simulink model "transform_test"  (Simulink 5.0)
settings: Solver=ode45  StartTime=0.0  StopTime=10.0  RelTol=1e-3
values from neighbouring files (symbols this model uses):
  a1 = 8.5    [startup.m]
  a2 = 48    [startup.m]
  a3 = 38+11/16    (= 38.6875)    [startup.m]
  a4 = 18.5    [startup.m]
  R1A = 10    [startup.m]
  R1B = 35.875    [startup.m]
  R2C = 36    [startup.m]
  R2D = 9+7/8    (= 9.875)    [startup.m]
  R3F = 4.5    [startup.m]
  R3G = 5.5    [startup.m]
  REF = 29.625    [startup.m]
  RFH = 9.5    [startup.m]
  RGH = 9.5    [startup.m]
  T01A = acos(RAJ/R1A)    [startup.m]
  T12C = acos((a2^2 + R2C^2 - R1C^2)/(2*a2*R2C))    [startup.m]
  T23D = 0.1317    [startup.m]
  TB12 = acos((R1B^2 + a2^2 - R2B^2)/(2*a2*R1B))    [startup.m]
  TD23 = acos((R2D^2 + a3^2 - R3D^2)/(2*a3*R2D))    [startup.m]
  TDFE = 0.0503    [startup.m]
  TG34 = 1.6966    [startup.m]
libraries: simulink x2

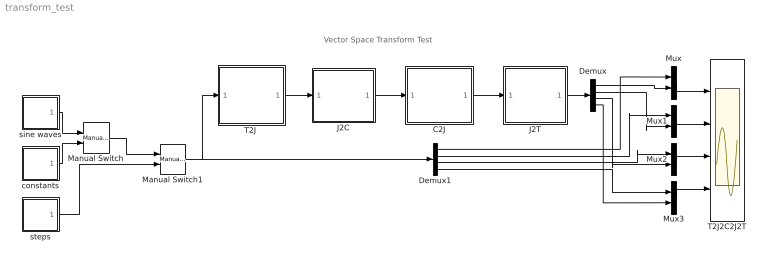
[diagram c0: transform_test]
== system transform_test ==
  note: Vector Space Transform Test
  C2J : Subsystem
  Demux : Demux
  Demux1 : Demux
  J2C : Subsystem
  J2T : Subsystem
  Manual Switch : simulink/Signal Routing/Manual Switch  sw=1  action=0
  Manual Switch1 : simulink/Signal Routing/Manual Switch  sw=1  action=0
  Mux{,1..3} (4 alike) : Mux  Inputs=2
  "T2J " : Subsystem
  T2J2C2J2T : Scope  NumInputPorts=4
  constants : Subsystem
  sine waves : Subsystem
  steps : Subsystem
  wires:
  Mux/1 -> T2J2C2J2T/1
  Mux1/1 -> T2J2C2J2T/2
  Mux2/1 -> T2J2C2J2T/3
  Mux3/1 -> T2J2C2J2T/4
  Demux1/1 -> Mux/1
  Demux1/2 -> Mux1/1
  Demux1/3 -> Mux2/1
  Demux1/4 -> Mux3/1
  Demux/1 -> Mux/2
  Demux/2 -> Mux1/2
  Demux/3 -> Mux2/2
  Demux/4 -> Mux3/2
  sine waves/1(ref) -> Manual Switch/1
  constants/1(ref) -> Manual Switch/2
  steps/1(ref) -> Manual Switch1/2
  Manual Switch/1 -> Manual Switch1/1
  Manual Switch1/1 -> Demux1/1, "T2J "/1(yp)
  J2C/1(ycdes) -> C2J/1(yc)
  "T2J "/1(qdes) -> J2C/1(qdes)
  C2J/1(q) -> J2T/1(q)
  J2T/1(yb) -> Demux/1

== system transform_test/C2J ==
  note: Swing
  note: q1
  note: Cylinder to Joint Transformation
  yc : Inport
  Boom : Subsystem
  Bucket : Subsystem
  Demux : Demux
  Mux : Mux
  Stick : Subsystem
  q : Outport
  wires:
  Mux/1 -> q/1
  yc/1 -> Demux/1
  Boom/1(q2) -> Mux/2
  Demux/2 -> Boom/1(yc3)
  Demux/1 -> Mux/1
  Demux/3 -> Stick/1(yc4)
  Stick/1(q3) -> Mux/3
  Demux/4 -> Bucket/1(yc5)
  Bucket/1(q4) -> Mux/4

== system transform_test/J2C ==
  note: Joint Space -> Cylinder Space Transformation
  note: Swing Cylinders
  qdes : Inport
  Boom cylinder : Subsystem
  Bucket cylinder : Subsystem
  Demux : Demux
  Mux : Mux
  Stick cylinder : Subsystem
  overswing  protection : Saturate  UpperLimit=pi/3  LowerLimit=-pi/2
  ycdes : Outport
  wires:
  qdes/1 -> Demux/1
  Mux/1 -> ycdes/1
  Demux/2 -> Boom cylinder/1(q2)
  Boom cylinder/1(yc3) -> Mux/2
  Demux/3 -> Stick cylinder/1(q3)
  Stick cylinder/1(yc4) -> Mux/3
  Demux/4 -> Bucket cylinder/1(q4)
  Bucket cylinder/1(yc5) -> Mux/4
  Demux/1 -> overswing  protection/1
  overswing  protection/1 -> Mux/1

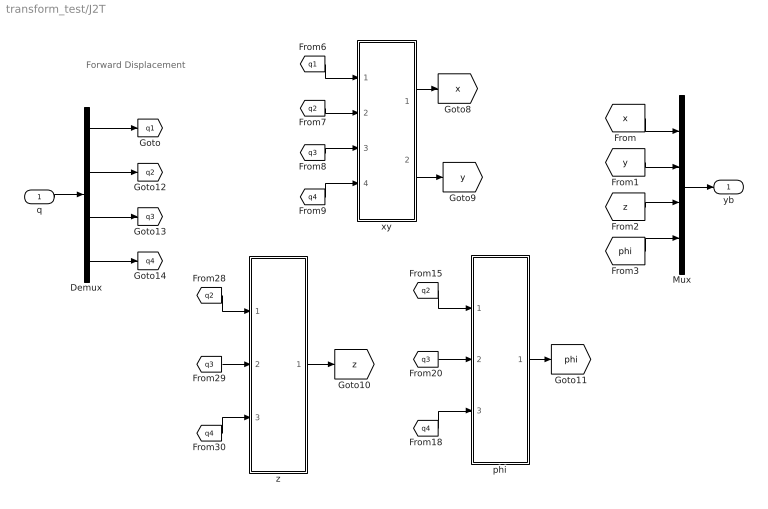
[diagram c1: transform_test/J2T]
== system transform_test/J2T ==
  note: Forward Displacement
  q : Inport
  Demux : Demux
  Mux : Mux
  phi : Subsystem
  xy : Subsystem
  z : Subsystem
  yb : Outport
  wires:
  [q2] -> z/1(q2)
  [q3] -> z/2(q3)
  [q4] -> z/3(q4)
  z/1(z) -> [z]
  q/1 -> Demux/1
  Demux/2 -> [q2]
  Demux/1 -> [q1]
  Demux/3 -> [q3]
  Demux/4 -> [q4]
  [q2] -> phi/1(q2)
  [q3] -> phi/2(q3)
  phi/1(phi) -> [phi]
  Mux/1 -> yb/1
  [x] -> Mux/1
  [y] -> Mux/2
  [z] -> Mux/3
  [phi] -> Mux/4
  xy/1(x) -> [x]
  [q1] -> xy/1(q1)
  [q2] -> xy/2(q2)
  [q3] -> xy/3(q3)
  [q4] -> xy/4(q4)
  [q4] -> phi/3(q4)
  xy/2(y) -> [y]

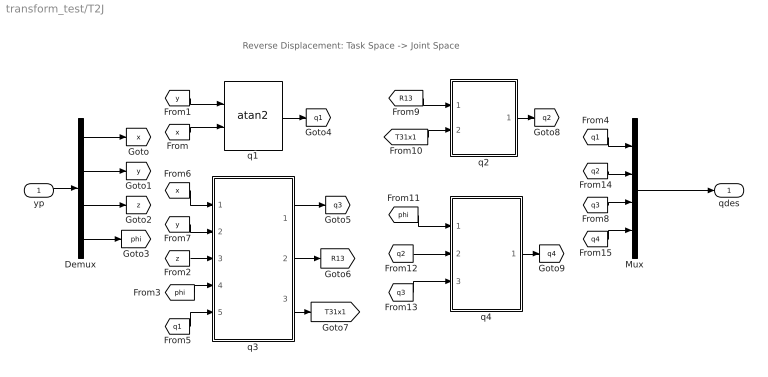
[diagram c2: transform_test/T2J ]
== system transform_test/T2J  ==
  note: Reverse Displacement: Task Space -> Joint Space
  yp : Inport
  Demux : Demux
  Mux : Mux
  q1 : Trigonometry  Operator=atan2
  q2 : Subsystem
  q3 : Subsystem
  q4 : Subsystem
  qdes : Outport
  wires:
  [x] -> q3/1(x)
  [y] -> q3/2(y)
  [z] -> q3/3(z)
  [phi] -> q3/4(phi)
  [q1] -> q3/5(q1)
  q3/1(q3) -> [q3]
  q3/2(R13) -> [R13]
  [y] -> q1/1
  [x] -> q1/2
  q1/1 -> [q1]
  q3/3(T31x1) -> [T31x1]
  [R13] -> q2/1(R13)
  [T31x1] -> q2/2(T31x1)
  [q3] -> q4/3(q3)
  [q2] -> q4/2(q2)
  [phi] -> q4/1(phi)
  q2/1(q2) -> [q2]
  q4/1(q4) -> [q4]
  Mux/1 -> qdes/1
  [q1] -> Mux/1
  [q3] -> Mux/3
  [q2] -> Mux/2
  [q4] -> Mux/4
  yp/1 -> Demux/1
  Demux/1 -> [x]
  Demux/2 -> [y]
  Demux/3 -> [z]
  Demux/4 -> [phi]

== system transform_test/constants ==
  DOF1 : Constant  Value=60
  DOF2 : Constant  Value=0
  DOF3 : Constant  Value=3
  DOF4 : Constant  Value=5*pi/6
  Mux2 : Mux
  ref : Outport
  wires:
  Mux2/1 -> ref/1
  DOF1/1 -> Mux2/1
  DOF2/1 -> Mux2/2
  DOF3/1 -> Mux2/3
  DOF4/1 -> Mux2/4

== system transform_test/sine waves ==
  DOF1 : Sin  Amplitude=4  Bias=46  Frequency=2*pi*0.1  SampleTime=0
  DOF2 : Sin  Amplitude=2  Frequency=2*pi*0.1  SampleTime=0
  DOF3 : Sin  Amplitude=6  Bias=3  Frequency=2*pi*0.1  SampleTime=0
  DOF4 : Sin  Amplitude=0.2  Bias=5*pi/6  Frequency=2*pi*0.1  SampleTime=0
  Mux2 : Mux
  ref : Outport
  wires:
  DOF1/1 -> Mux2/1
  DOF4/1 -> Mux2/4
  DOF3/1 -> Mux2/3
  DOF2/1 -> Mux2/2
  Mux2/1 -> ref/1

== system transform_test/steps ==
  Constant : Constant  Value=[46 0 3 5*pi/6]
  DOF1 : Step  Time=0.25  SampleTime=0
  DOF2 : Step  Time=0.5  After=0.5  SampleTime=0
  DOF3 : Step  Time=.75  After=-.5  SampleTime=0
  DOF4 : Step  After=-1  SampleTime=0
  Mux2 : Mux
  Sum : Sum  Inputs=|++
  ref : Outport
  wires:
  DOF1/1 -> Mux2/1
  DOF4/1 -> Mux2/4
  DOF3/1 -> Mux2/3
  DOF2/1 -> Mux2/2
  Mux2/1 -> Sum/1
  Sum/1 -> ref/1
  Constant/1 -> Sum/2

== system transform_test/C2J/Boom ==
  note: TA1B
  yc3 : Inport
  CosineLawA : Subsystem
  R1A : Constant  Value=R1A
  R1B : Constant  Value=R1B
  Sum : Sum  Inputs=+---
  T01A : Constant  Value=T01A
  TA1B : Constant  Value=TB12
  pi : Constant  Value=pi
  q2 : Outport
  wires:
  pi/1 -> Sum/1
  T01A/1 -> Sum/2
  TA1B/1 -> Sum/4
  CosineLawA/1(theta) -> Sum/3
  R1A/1 -> CosineLawA/1(r1)
  R1B/1 -> CosineLawA/2(r2)
  Sum/1 -> q2/1
  yc3/1 -> CosineLawA/3(r3)

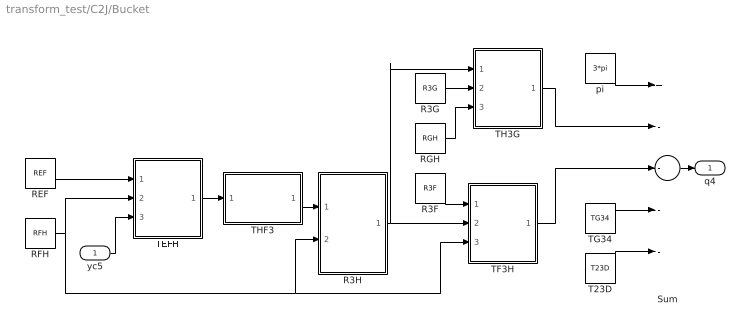
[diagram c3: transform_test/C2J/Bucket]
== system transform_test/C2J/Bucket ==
  yc5 : Inport
  R3F : Constant  Value=R3F
  R3G : Constant  Value=R3G
  R3H : Subsystem
  REF : Constant  Value=REF
  RFH : Constant  Value=RFH
  RGH : Constant  Value=RGH
  Sum : Sum  Inputs=+----
  T23D : Constant  Value=T23D
  TEFH : Subsystem
  TF3H : Subsystem
  TG34 : Constant  Value=TG34
  TH3G : Subsystem
  THF3 : Subsystem
  pi : Constant  Value=3*pi
  q4 : Outport
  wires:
  TEFH/1(TEFH) -> THF3/1(TEFH)
  REF/1 -> TEFH/1(r1)
  yc5/1 -> TEFH/3(r3)
  RFH/1 -> TEFH/2(r2), R3H/2(RFH), TF3H/3(r3)
  THF3/1(THF3) -> R3H/1(THF3)
  R3F/1 -> TF3H/1(r1)
  R3H/1(R3H) -> TF3H/2(r2), TH3G/1(r1)
  R3G/1 -> TH3G/2(r2)
  RGH/1 -> TH3G/3(r3)
  pi/1 -> Sum/1
  Sum/1 -> q4/1
  T23D/1 -> Sum/5
  TG34/1 -> Sum/4
  TH3G/1(TH3G) -> Sum/2
  TF3H/1(TF3H) -> Sum/3

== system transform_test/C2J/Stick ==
  note: TC2D
  yc4 : Inport
  CosineLawA : Subsystem
  R2C : Constant  Value=R2C
  R2D : Constant  Value=R2D
  Sum : Sum  Inputs=+---
  T12C : Constant  Value=T12C
  TD23 : Constant  Value=TD23
  pi : Constant  Value=3*pi
  q3 : Outport
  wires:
  pi/1 -> Sum/1
  T12C/1 -> Sum/2
  TD23/1 -> Sum/4
  CosineLawA/1(theta) -> Sum/3
  R2C/1 -> CosineLawA/1(r1)
  R2D/1 -> CosineLawA/2(r2)
  Sum/1 -> q3/1
  yc4/1 -> CosineLawA/3(r3)

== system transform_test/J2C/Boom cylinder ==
  q2 : Inport
  Constant : Constant  Value=pi
  Constant1 : Constant  Value=T01A
  Constant2 : Constant  Value=TB12
  CosineLawB : Subsystem
  Sum : Sum  Inputs=+---
  yc3 : Outport
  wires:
  Constant/1 -> Sum/1
  Constant1/1 -> Sum/2
  Sum/1 -> CosineLawB/1(TA1B)
  CosineLawB/1(yc3) -> yc3/1
  q2/1 -> Sum/3
  Constant2/1 -> Sum/4

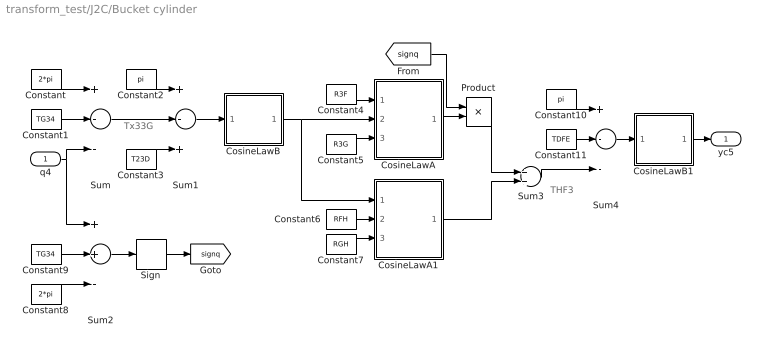
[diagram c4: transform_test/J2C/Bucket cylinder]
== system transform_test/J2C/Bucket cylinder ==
  note: Tx33G
  note: THF3
  q4 : Inport
  Constant : Constant  Value=2*pi
  Constant1 : Constant  Value=TG34
  Constant10 : Constant  Value=pi
  Constant11 : Constant  Value=TDFE
  Constant2 : Constant  Value=pi
  Constant3 : Constant  Value=T23D
  Constant4 : Constant  Value=R3F
  Constant5 : Constant  Value=R3G
  Constant6 : Constant  Value=RFH
  Constant7 : Constant  Value=RGH
  Constant8 : Constant  Value=2*pi
  Constant9 : Constant  Value=TG34
  CosineLawA : Subsystem
  CosineLawA1 : Subsystem
  CosineLawB : Subsystem
  CosineLawB1 : Subsystem
  Product : Product
  Sign : Signum
  Sum : Sum  Inputs=+--
  Sum1 : Sum  Inputs=+-+
  Sum2 : Sum  Inputs=++-
  Sum3 : Sum
  Sum4 : Sum  Inputs=+--
  yc5 : Outport
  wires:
  Constant/1 -> Sum/1
  Constant1/1 -> Sum/2
  Sum/1 -> Sum1/2
  Constant2/1 -> Sum1/1
  Constant3/1 -> Sum1/3
  Sum1/1 -> CosineLawB/1(TG3F)
  CosineLawB/1(rFG) -> CosineLawA/2(r2), CosineLawA1/1(r1)
  Constant4/1 -> CosineLawA/1(r1)
  Constant5/1 -> CosineLawA/3(r3)
  Constant6/1 -> CosineLawA1/2(r2)
  Constant7/1 -> CosineLawA1/3(r3)
  Constant9/1 -> Sum2/2
  Constant8/1 -> Sum2/3
  Sum2/1 -> Sign/1
  [signq] -> Product/1
  CosineLawA/1(T3FG) -> Product/2
  Sign/1 -> [signq]
  Product/1 -> Sum3/1
  CosineLawA1/1(THFG) -> Sum3/2
  Constant10/1 -> Sum4/1
  Sum3/1 -> Sum4/3
  Constant11/1 -> Sum4/2
  Sum4/1 -> CosineLawB1/1(TEFH)
  CosineLawB1/1(yc5) -> yc5/1
  q4/1 -> Sum/3, Sum2/1

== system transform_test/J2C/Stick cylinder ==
  q3 : Inport
  Constant : Constant  Value=pi
  Constant1 : Constant  Value=TD23
  Constant2 : Constant  Value=T12C
  CosineLawB : Subsystem
  Sum : Sum  Inputs=+---
  yc4 : Outport
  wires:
  Constant/1 -> Sum/1
  Constant1/1 -> Sum/2
  Sum/1 -> CosineLawB/1(TC2D)
  CosineLawB/1(yc4) -> yc4/1
  q3/1 -> Sum/3
  Constant2/1 -> Sum/4

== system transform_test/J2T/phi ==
  q2 : Inport
  q3 : Inport  Port=2
  q4 : Inport  Port=3
  Constant : Constant  Value=3*pi
  Sum : Sum  Inputs=+++-
  phi : Outport
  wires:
  q2/1 -> Sum/1
  q3/1 -> Sum/2
  q4/1 -> Sum/3
  Constant/1 -> Sum/4
  Sum/1 -> phi/1

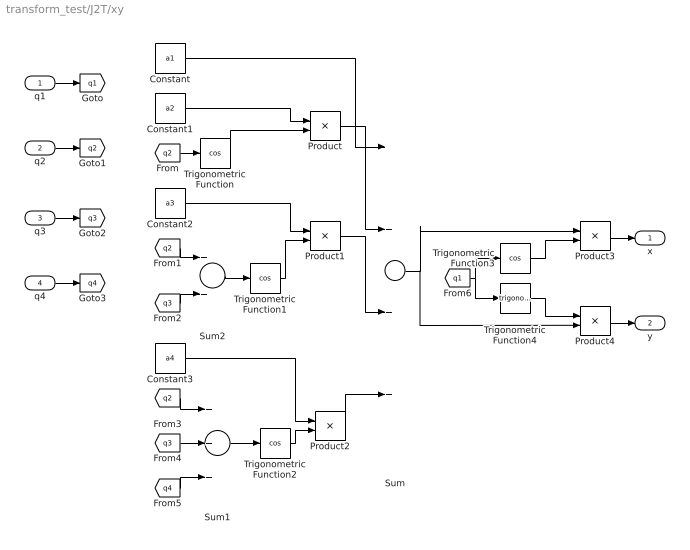
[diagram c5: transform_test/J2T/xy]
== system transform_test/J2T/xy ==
  q1 : Inport
  q2 : Inport  Port=2
  q3 : Inport  Port=3
  q4 : Inport  Port=4
  Constant : Constant  Value=a1
  Constant1 : Constant  Value=a2
  Constant2 : Constant  Value=a3
  Constant3 : Constant  Value=a4
  Product{,1..4} (5 alike) : Product
  Sum : Sum  Inputs=++++
  Sum1 : Sum  Inputs=+++
  Sum2 : Sum
  Trigonometric Function{,1..3} (4 alike) : Trigonometry  Operator=cos
  Trigonometric Function4 : Trigonometry
  x : Outport
  y : Outport  Port=2
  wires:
  q1/1 -> [q1]
  q2/1 -> [q2]
  q3/1 -> [q3]
  q4/1 -> [q4]
  Constant/1 -> Sum/1
  Product/1 -> Sum/2
  Constant1/1 -> Product/1
  [q3] -> Sum2/2
  [q2] -> Sum2/1
  Constant2/1 -> Product1/1
  Product1/1 -> Sum/3
  Product2/1 -> Sum/4
  Constant3/1 -> Product2/1
  [q2] -> Sum1/1
  [q3] -> Sum1/2
  [q4] -> Sum1/3
  Product3/1 -> x/1
  Sum/1 -> Product4/2, Product3/1
  Trigonometric Function/1 -> Product/2
  [q2] -> Trigonometric Function/1
  Sum2/1 -> Trigonometric Function1/1
  Trigonometric Function1/1 -> Product1/2
  Sum1/1 -> Trigonometric Function2/1
  Trigonometric Function2/1 -> Product2/2
  Product4/1 -> y/1
  Trigonometric Function3/1 -> Product3/2
  [q1] -> Trigonometric Function3/1, Trigonometric Function4/1
  Trigonometric Function4/1 -> Product4/1

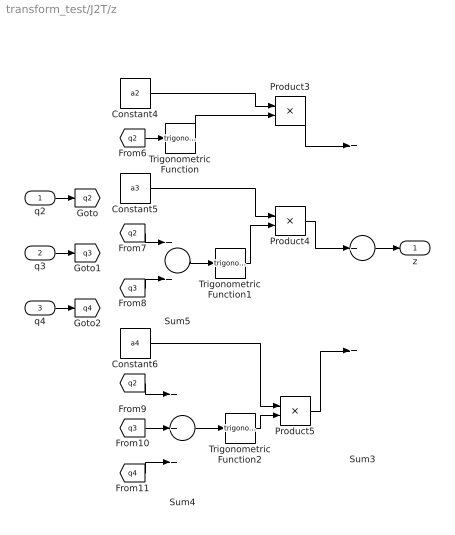
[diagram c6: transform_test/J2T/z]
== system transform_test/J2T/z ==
  q2 : Inport
  q3 : Inport  Port=2
  q4 : Inport  Port=3
  Constant4 : Constant  Value=a2
  Constant5 : Constant  Value=a3
  Constant6 : Constant  Value=a4
  Product3 : Product
  Product4 : Product
  Product5 : Product
  Sum3 : Sum  Inputs=+++
  Sum4 : Sum  Inputs=+++
  Sum5 : Sum
  Trigonometric Function : Trigonometry
  Trigonometric Function1 : Trigonometry
  Trigonometric Function2 : Trigonometry
  z : Outport
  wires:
  q3/1 -> [q3]
  q4/1 -> [q4]
  q2/1 -> [q2]
  Constant4/1 -> Product3/1
  [q3] -> Sum5/2
  [q2] -> Sum5/1
  Constant5/1 -> Product4/1
  Constant6/1 -> Product5/1
  [q2] -> Sum4/1
  [q3] -> Sum4/2
  [q4] -> Sum4/3
  Trigonometric Function/1 -> Product3/2
  [q2] -> Trigonometric Function/1
  Sum5/1 -> Trigonometric Function1/1
  Trigonometric Function1/1 -> Product4/2
  Sum4/1 -> Trigonometric Function2/1
  Trigonometric Function2/1 -> Product5/2
  Product3/1 -> Sum3/1
  Product4/1 -> Sum3/2
  Product5/1 -> Sum3/3
  Sum3/1 -> z/1

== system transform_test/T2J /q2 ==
  note: T213
  R13 : Inport
  T31x1 : Inport  Port=2
  CosineLawA : Subsystem
  Sum : Sum  Inputs=|++
  a2 : Constant  Value=a2
  a3 : Constant  Value=a3
  q2 : Outport
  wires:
  a2/1 -> CosineLawA/1(r1)
  a3/1 -> CosineLawA/3(r3)
  CosineLawA/1(theta) -> Sum/1
  Sum/1 -> q2/1
  R13/1 -> CosineLawA/2(r2)
  T31x1/1 -> Sum/2

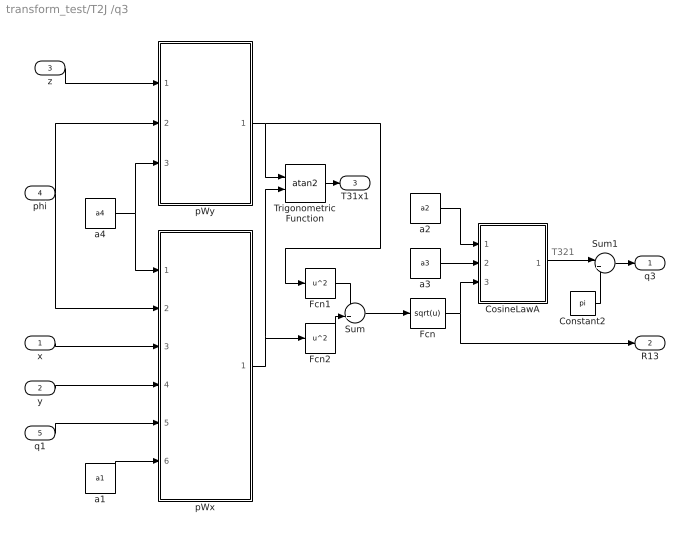
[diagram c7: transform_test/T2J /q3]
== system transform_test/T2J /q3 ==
  note: T321
  x : Inport
  y : Inport  Port=2
  z : Inport  Port=3
  phi : Inport  Port=4
  q1 : Inport  Port=5
  Constant2 : Constant  Value=pi
  CosineLawA : Subsystem
  Fcn : Fcn  Expr=sqrt(u)
  Fcn1 : Fcn  Expr=u^2
  Fcn2 : Fcn  Expr=u^2
  Sum : Sum
  Sum1 : Sum  Inputs=|++
  Trigonometric Function : Trigonometry  Operator=atan2
  a1 : Constant  Value=a1
  a2 : Constant  Value=a2
  a3 : Constant  Value=a3
  a4 : Constant  Value=a4
  pWx : Subsystem
  pWy : Subsystem
  q3 : Outport
  R13 : Outport  Port=2
  T31x1 : Outport  Port=3
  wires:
  a1/1 -> pWx/6(a1)
  q1/1 -> pWx/5(q1)
  y/1 -> pWx/4(y)
  x/1 -> pWx/3(x)
  a4/1 -> pWx/1(a4), pWy/3(a4)
  z/1 -> pWy/1(z)
  phi/1 -> pWx/2(phi), pWy/2(phi)
  pWy/1(pWy) -> Fcn1/1, Trigonometric Function/1
  Trigonometric Function/1 -> T31x1/1
  Fcn1/1 -> Sum/1
  Fcn2/1 -> Sum/2
  Sum/1 -> Fcn/1
  pWx/1(pWx) -> Fcn2/1, Trigonometric Function/2
  a3/1 -> CosineLawA/2(r2)
  a2/1 -> CosineLawA/1(r1)
  Fcn/1 -> CosineLawA/3(r3), R13/1
  Sum1/1 -> q3/1
  Constant2/1 -> Sum1/2
  CosineLawA/1(theta) -> Sum1/1

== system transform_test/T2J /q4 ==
  phi : Inport
  q2 : Inport  Port=2
  q3 : Inport  Port=3
  Constant : Constant  Value=3*pi
  Sum : Sum  Inputs=+--+
  q4 : Outport
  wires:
  phi/1 -> Sum/1
  q2/1 -> Sum/2
  Sum/1 -> q4/1
  q3/1 -> Sum/3
  Constant/1 -> Sum/4

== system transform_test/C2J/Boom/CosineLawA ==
  r1 : Inport
  r2 : Inport  Port=2
  r3 : Inport  Port=3
  Fcn1 : Fcn  Expr=u^2
  Fcn2 : Fcn  Expr=u^2
  Fcn3 : Fcn  Expr=u^2
  Gain : Gain  Gain=2
  Product : Product
  Product1 : Product  Inputs=*/
  Sum : Sum  Inputs=++-
  Trigonometric Function : Trigonometry  Operator=acos
  theta : Outport
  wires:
  r3/1 -> Fcn3/1
  Fcn1/1 -> Sum/1
  Fcn2/1 -> Sum/2
  Fcn3/1 -> Sum/3
  r2/1 -> Fcn2/1, Product/1
  r1/1 -> Fcn1/1, Product/2
  Product/1 -> Gain/1
  Sum/1 -> Product1/1
  Gain/1 -> Product1/2
  Product1/1 -> Trigonometric Function/1
  Trigonometric Function/1 -> theta/1

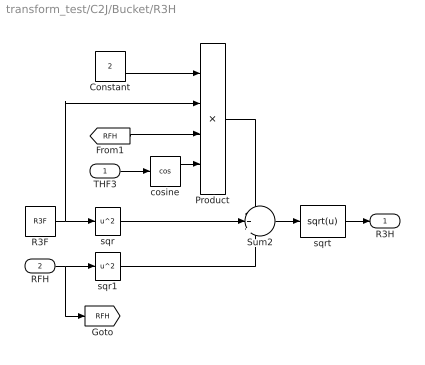
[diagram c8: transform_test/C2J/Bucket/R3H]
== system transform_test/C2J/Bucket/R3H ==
  THF3 : Inport
  RFH : Inport  Port=2
  Constant : Constant  Value=2
  Product : Product  Inputs=4
  R3F : Constant  Value=R3F
  Sum2 : Sum  Inputs=-++
  cosine : Trigonometry  Operator=cos
  sqr : Fcn  Expr=u^2
  sqr1 : Fcn  Expr=u^2
  sqrt : Fcn  Expr=sqrt(u)
  R3H : Outport
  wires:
  R3F/1 -> sqr/1, Product/2
  sqr1/1 -> Sum2/3
  Constant/1 -> Product/1
  [RFH] -> Product/3
  sqr/1 -> Sum2/2
  Product/1 -> Sum2/1
  cosine/1 -> Product/4
  Sum2/1 -> sqrt/1
  THF3/1 -> cosine/1
  sqrt/1 -> R3H/1
  RFH/1 -> sqr1/1, [RFH]

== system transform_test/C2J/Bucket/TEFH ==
  r1 : Inport
  r2 : Inport  Port=2
  r3 : Inport  Port=3
  Fcn1 : Fcn  Expr=u^2
  Fcn2 : Fcn  Expr=u^2
  Fcn3 : Fcn  Expr=u^2
  Gain : Gain  Gain=2
  Product : Product
  Product1 : Product  Inputs=*/
  Sum : Sum  Inputs=++-
  Trigonometric Function : Trigonometry  Operator=acos
  TEFH : Outport
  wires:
  r3/1 -> Fcn3/1
  Fcn1/1 -> Sum/1
  Fcn2/1 -> Sum/2
  Fcn3/1 -> Sum/3
  r2/1 -> Fcn2/1, Product/1
  r1/1 -> Fcn1/1, Product/2
  Product/1 -> Gain/1
  Sum/1 -> Product1/1
  Gain/1 -> Product1/2
  Product1/1 -> Trigonometric Function/1
  Trigonometric Function/1 -> TEFH/1

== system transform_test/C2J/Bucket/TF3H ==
  r1 : Inport
  r2 : Inport  Port=2
  r3 : Inport  Port=3
  Fcn1 : Fcn  Expr=u^2
  Fcn2 : Fcn  Expr=u^2
  Fcn3 : Fcn  Expr=u^2
  Gain : Gain  Gain=2
  Product : Product
  Product1 : Product  Inputs=*/
  Sum : Sum  Inputs=++-
  Trigonometric Function : Trigonometry  Operator=acos
  TF3H : Outport
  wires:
  r3/1 -> Fcn3/1
  Fcn1/1 -> Sum/1
  Fcn2/1 -> Sum/2
  Fcn3/1 -> Sum/3
  r2/1 -> Fcn2/1, Product/1
  r1/1 -> Fcn1/1, Product/2
  Product/1 -> Gain/1
  Sum/1 -> Product1/1
  Gain/1 -> Product1/2
  Product1/1 -> Trigonometric Function/1
  Trigonometric Function/1 -> TF3H/1

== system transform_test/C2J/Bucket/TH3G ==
  r1 : Inport
  r2 : Inport  Port=2
  r3 : Inport  Port=3
  Fcn1 : Fcn  Expr=u^2
  Fcn2 : Fcn  Expr=u^2
  Fcn3 : Fcn  Expr=u^2
  Gain : Gain  Gain=2
  Product : Product
  Product1 : Product  Inputs=*/
  Sum : Sum  Inputs=++-
  Trigonometric Function : Trigonometry  Operator=acos
  TH3G : Outport
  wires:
  r3/1 -> Fcn3/1
  Fcn1/1 -> Sum/1
  Fcn2/1 -> Sum/2
  Fcn3/1 -> Sum/3
  r2/1 -> Fcn2/1, Product/1
  r1/1 -> Fcn1/1, Product/2
  Product/1 -> Gain/1
  Sum/1 -> Product1/1
  Gain/1 -> Product1/2
  Product1/1 -> Trigonometric Function/1
  Trigonometric Function/1 -> TH3G/1

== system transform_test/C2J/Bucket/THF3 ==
  TEFH : Inport
  Sum1 : Sum  Inputs=+--
  TDFE : Constant  Value=TDFE
  pi1 : Constant  Value=pi
  THF3 : Outport
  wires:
  pi1/1 -> Sum1/1
  TDFE/1 -> Sum1/2
  Sum1/1 -> THF3/1
  TEFH/1 -> Sum1/3

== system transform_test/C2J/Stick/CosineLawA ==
  r1 : Inport
  r2 : Inport  Port=2
  r3 : Inport  Port=3
  Fcn1 : Fcn  Expr=u^2
  Fcn2 : Fcn  Expr=u^2
  Fcn3 : Fcn  Expr=u^2
  Gain : Gain  Gain=2
  Product : Product
  Product1 : Product  Inputs=*/
  Sum : Sum  Inputs=++-
  Trigonometric Function : Trigonometry  Operator=acos
  theta : Outport
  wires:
  r3/1 -> Fcn3/1
  Fcn1/1 -> Sum/1
  Fcn2/1 -> Sum/2
  Fcn3/1 -> Sum/3
  r2/1 -> Fcn2/1, Product/1
  r1/1 -> Fcn1/1, Product/2
  Product/1 -> Gain/1
  Sum/1 -> Product1/1
  Gain/1 -> Product1/2
  Product1/1 -> Trigonometric Function/1
  Trigonometric Function/1 -> theta/1

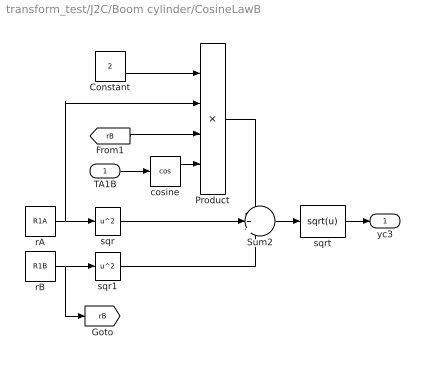
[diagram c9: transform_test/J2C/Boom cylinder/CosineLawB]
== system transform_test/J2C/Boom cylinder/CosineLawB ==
  TA1B : Inport
  Constant : Constant  Value=2
  Product : Product  Inputs=4
  Sum2 : Sum  Inputs=-++
  cosine : Trigonometry  Operator=cos
  rA : Constant  Value=R1A
  rB : Constant  Value=R1B
  sqr : Fcn  Expr=u^2
  sqr1 : Fcn  Expr=u^2
  sqrt : Fcn  Expr=sqrt(u)
  yc3 : Outport
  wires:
  rA/1 -> sqr/1, Product/2
  sqr1/1 -> Sum2/3
  Constant/1 -> Product/1
  [rB] -> Product/3
  sqr/1 -> Sum2/2
  Product/1 -> Sum2/1
  cosine/1 -> Product/4
  Sum2/1 -> sqrt/1
  TA1B/1 -> cosine/1
  sqrt/1 -> yc3/1
  rB/1 -> sqr1/1, [rB]

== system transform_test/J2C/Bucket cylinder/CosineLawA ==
  r1 : Inport
  r2 : Inport  Port=2
  r3 : Inport  Port=3
  Fcn1 : Fcn  Expr=u^2
  Fcn2 : Fcn  Expr=u^2
  Fcn3 : Fcn  Expr=u^2
  Gain : Gain  Gain=2
  Product : Product
  Product1 : Product  Inputs=*/
  Sum : Sum  Inputs=++-
  Trigonometric Function : Trigonometry  Operator=acos
  T3FG : Outport
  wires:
  r3/1 -> Fcn3/1
  Fcn1/1 -> Sum/1
  Fcn2/1 -> Sum/2
  Fcn3/1 -> Sum/3
  r2/1 -> Fcn2/1, Product/1
  r1/1 -> Fcn1/1, Product/2
  Product/1 -> Gain/1
  Sum/1 -> Product1/1
  Gain/1 -> Product1/2
  Product1/1 -> Trigonometric Function/1
  Trigonometric Function/1 -> T3FG/1

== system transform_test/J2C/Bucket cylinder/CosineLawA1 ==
  r1 : Inport
  r2 : Inport  Port=2
  r3 : Inport  Port=3
  Fcn1 : Fcn  Expr=u^2
  Fcn2 : Fcn  Expr=u^2
  Fcn3 : Fcn  Expr=u^2
  Gain : Gain  Gain=2
  Product : Product
  Product1 : Product  Inputs=*/
  Sum : Sum  Inputs=++-
  Trigonometric Function : Trigonometry  Operator=acos
  THFG : Outport
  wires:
  r3/1 -> Fcn3/1
  Fcn1/1 -> Sum/1
  Fcn2/1 -> Sum/2
  Fcn3/1 -> Sum/3
  r2/1 -> Fcn2/1, Product/1
  r1/1 -> Fcn1/1, Product/2
  Product/1 -> Gain/1
  Sum/1 -> Product1/1
  Gain/1 -> Product1/2
  Product1/1 -> Trigonometric Function/1
  Trigonometric Function/1 -> THFG/1

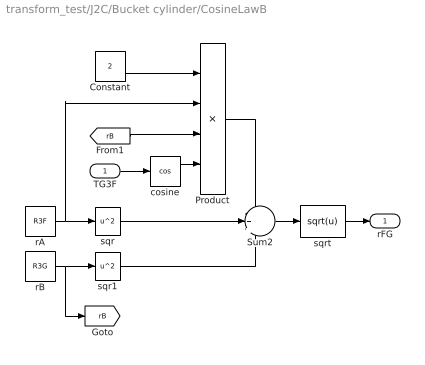
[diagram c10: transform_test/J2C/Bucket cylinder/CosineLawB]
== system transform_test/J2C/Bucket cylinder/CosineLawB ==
  TG3F : Inport
  Constant : Constant  Value=2
  Product : Product  Inputs=4
  Sum2 : Sum  Inputs=-++
  cosine : Trigonometry  Operator=cos
  rA : Constant  Value=R3F
  rB : Constant  Value=R3G
  sqr : Fcn  Expr=u^2
  sqr1 : Fcn  Expr=u^2
  sqrt : Fcn  Expr=sqrt(u)
  rFG : Outport
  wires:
  rA/1 -> sqr/1, Product/2
  sqr1/1 -> Sum2/3
  Constant/1 -> Product/1
  [rB] -> Product/3
  sqr/1 -> Sum2/2
  Product/1 -> Sum2/1
  cosine/1 -> Product/4
  Sum2/1 -> sqrt/1
  TG3F/1 -> cosine/1
  sqrt/1 -> rFG/1
  rB/1 -> sqr1/1, [rB]

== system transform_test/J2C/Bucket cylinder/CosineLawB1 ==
  TEFH : Inport
  Constant : Constant  Value=2
  Product : Product  Inputs=4
  Sum2 : Sum  Inputs=-++
  cosine : Trigonometry  Operator=cos
  rA : Constant  Value=REF
  rB : Constant  Value=RFH
  sqr : Fcn  Expr=u^2
  sqr1 : Fcn  Expr=u^2
  sqrt : Fcn  Expr=sqrt(u)
  yc5 : Outport
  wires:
  rA/1 -> sqr/1, Product/2
  sqr1/1 -> Sum2/3
  Constant/1 -> Product/1
  [rB] -> Product/3
  sqr/1 -> Sum2/2
  Product/1 -> Sum2/1
  cosine/1 -> Product/4
  Sum2/1 -> sqrt/1
  TEFH/1 -> cosine/1
  sqrt/1 -> yc5/1
  rB/1 -> sqr1/1, [rB]

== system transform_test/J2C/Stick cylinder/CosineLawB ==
  TC2D : Inport
  Constant : Constant  Value=2
  Product : Product  Inputs=4
  Sum2 : Sum  Inputs=-++
  cosine : Trigonometry  Operator=cos
  rA : Constant  Value=R2C
  rB : Constant  Value=R2D
  sqr : Fcn  Expr=u^2
  sqr1 : Fcn  Expr=u^2
  sqrt : Fcn  Expr=sqrt(u)
  yc4 : Outport
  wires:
  rA/1 -> sqr/1, Product/2
  sqr1/1 -> Sum2/3
  Constant/1 -> Product/1
  [rB] -> Product/3
  sqr/1 -> Sum2/2
  Product/1 -> Sum2/1
  cosine/1 -> Product/4
  Sum2/1 -> sqrt/1
  TC2D/1 -> cosine/1
  sqrt/1 -> yc4/1
  rB/1 -> sqr1/1, [rB]

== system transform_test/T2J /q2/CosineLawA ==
  r1 : Inport
  r2 : Inport  Port=2
  r3 : Inport  Port=3
  Fcn1 : Fcn  Expr=u^2
  Fcn2 : Fcn  Expr=u^2
  Fcn3 : Fcn  Expr=u^2
  Gain : Gain  Gain=2
  Product : Product
  Product1 : Product  Inputs=*/
  Sum : Sum  Inputs=++-
  Trigonometric Function : Trigonometry  Operator=acos
  theta : Outport
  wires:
  r3/1 -> Fcn3/1
  Fcn1/1 -> Sum/1
  Fcn2/1 -> Sum/2
  Fcn3/1 -> Sum/3
  r2/1 -> Fcn2/1, Product/1
  r1/1 -> Fcn1/1, Product/2
  Product/1 -> Gain/1
  Sum/1 -> Product1/1
  Gain/1 -> Product1/2
  Product1/1 -> Trigonometric Function/1
  Trigonometric Function/1 -> theta/1

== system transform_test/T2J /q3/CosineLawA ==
  r1 : Inport
  r2 : Inport  Port=2
  r3 : Inport  Port=3
  Fcn1 : Fcn  Expr=u^2
  Fcn2 : Fcn  Expr=u^2
  Fcn3 : Fcn  Expr=u^2
  Gain : Gain  Gain=2
  Product : Product
  Product1 : Product  Inputs=*/
  Sum : Sum  Inputs=++-
  Trigonometric Function : Trigonometry  Operator=acos
  theta : Outport
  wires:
  r3/1 -> Fcn3/1
  Fcn1/1 -> Sum/1
  Fcn2/1 -> Sum/2
  Fcn3/1 -> Sum/3
  r2/1 -> Fcn2/1, Product/1
  r1/1 -> Fcn1/1, Product/2
  Product/1 -> Gain/1
  Sum/1 -> Product1/1
  Gain/1 -> Product1/2
  Product1/1 -> Trigonometric Function/1
  Trigonometric Function/1 -> theta/1

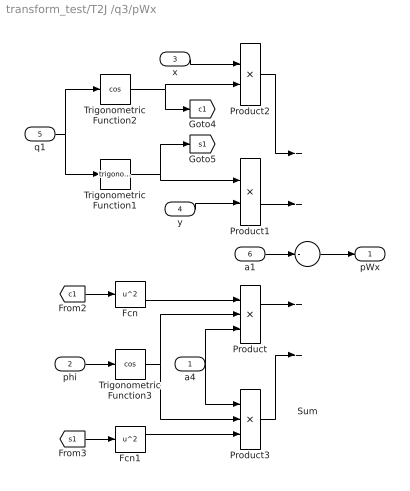
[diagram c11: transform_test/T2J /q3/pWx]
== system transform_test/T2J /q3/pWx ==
  a4 : Inport
  phi : Inport  Port=2
  x : Inport  Port=3
  y : Inport  Port=4
  q1 : Inport  Port=5
  a1 : Inport  Port=6
  Fcn : Fcn  Expr=u^2
  Fcn1 : Fcn  Expr=u^2
  Product : Product  Inputs=3
  Product1 : Product
  Product2 : Product
  Product3 : Product  Inputs=3
  Sum : Sum  Inputs=++-++
  Trigonometric Function1 : Trigonometry
  Trigonometric Function2 : Trigonometry  Operator=cos
  Trigonometric Function3 : Trigonometry  Operator=cos
  pWx : Outport
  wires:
  Product2/1 -> Sum/1
  Product1/1 -> Sum/2
  x/1 -> Product2/1
  Sum/1 -> pWx/1
  a1/1 -> Sum/3
  q1/1 -> Trigonometric Function2/1, Trigonometric Function1/1
  y/1 -> Product1/2
  Trigonometric Function1/1 -> Product1/1, [s1]
  Trigonometric Function2/1 -> Product2/2, [c1]
  Product/1 -> Sum/4
  Product3/1 -> Sum/5
  [c1] -> Fcn/1
  Fcn/1 -> Product/1
  a4/1 -> Product/3, Product3/1
  Trigonometric Function3/1 -> Product/2, Product3/2
  Fcn1/1 -> Product3/3
  [s1] -> Fcn1/1
  phi/1 -> Trigonometric Function3/1

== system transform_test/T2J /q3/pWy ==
  z : Inport
  phi : Inport  Port=2
  a4 : Inport  Port=3
  Product : Product
  Sum : Sum  Inputs=|++
  Trigonometric Function : Trigonometry
  pWy : Outport
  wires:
  Trigonometric Function/1 -> Product/2
  a4/1 -> Product/1
  Product/1 -> Sum/1
  Sum/1 -> pWy/1
  phi/1 -> Trigonometric Function/1
  z/1 -> Sum/2
